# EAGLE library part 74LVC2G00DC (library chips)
NAND, 2-Array
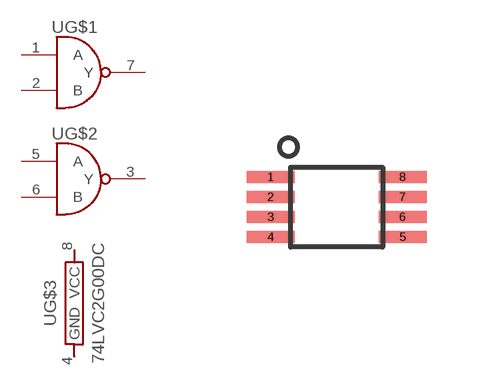
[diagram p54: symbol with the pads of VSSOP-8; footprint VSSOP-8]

Designator prefix U; gates G$1=NAND G$2=NAND G$3=SUPPLY

## 74LVC2G00DC (DIGIKEY: 568-7671-1-ND)  [VSSOP-8]
1  G$1:A
2  G$1:B
3  G$2:Y
4  G$3:GND
5  G$2:A
6  G$2:B
7  G$1:Y
8  G$3:VCC

## Footprint VSSOP-8 (pad centres in mm)
smd 1.2 x 0.3: 1 -1.65,0.75; 2 -1.65,0.25; 3 -1.65,-0.25; 4 -1.65,-0.75; 5 1.65,-0.75; 6 1.65,-0.25; 7 1.65,0.25; 8 1.65,0.75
